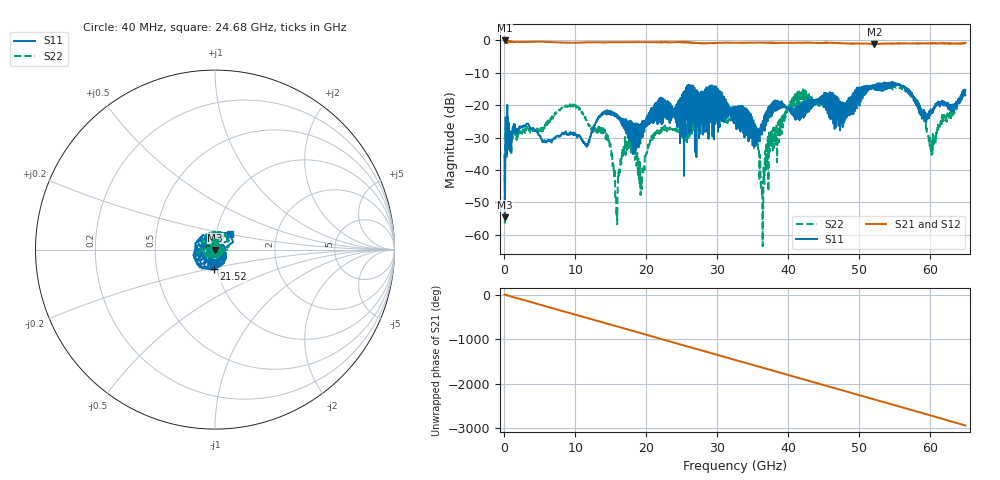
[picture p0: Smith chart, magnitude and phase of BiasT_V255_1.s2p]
! Created Tue Jul 15 19:49:57 2008
# hz S ma R 50
! 2 Port Network Data from blockName block
! freq  magS11  angS11  magS21  angS21  magS12  angS12  magS22  angS22
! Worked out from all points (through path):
!   1601 points, 40 MHz to 65 GHz, reference 50 ohm
!   highest |S21| = -0.03 dB at 80.6 MHz (marker M1); lowest = -1.1 dB at 52.17 GHz (marker M2)
!   group delay of S21, straight-line fit = 125 ps
!   lowest |S11| = -54.7 dB at 80.6 MHz (marker M3), VSWR 1.00, Z = 50.1 - j0.149 ohm
!   |S11| at or under -10 dB: start of sweep to end of sweep
!   |S22| runs from -63.5 to -13.2 dB; largest |S21 - S12| = 0.05
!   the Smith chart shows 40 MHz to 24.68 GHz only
!   S11 on the Smith chart (normalised r, x): 40 MHz: 1.00, +0.03; 21.52 GHz: 0.96, -0.21; 24.68 GHz: 1.16, +0.21
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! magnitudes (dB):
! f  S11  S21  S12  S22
! 40 MHz  -35.6  -0.1  -0.1  -35.2
! 80.6 MHz  -54.7  0.0  0.0  -56.9
! 3.085 GHz  -26.0  -0.5  -0.5  -27.5
! 10.88 GHz  -30.3  -0.7  -0.7  -21.8
! 14.45 GHz  -22.2  -0.6  -0.6  -30.7
! 15.75 GHz  -23.6  -0.6  -0.6  -48.2
! 17.09 GHz  -25.5  -0.6  -0.5  -35.4
! 19.32 GHz  -30.2  -0.5  -0.5  -42.5
! 21.52 GHz  -19.2  -0.6  -0.5  -28.0
! 21.72 GHz  -19.0  -0.6  -0.5  -27.7
! 24.68 GHz  -18.3  -0.6  -0.5  -27.9
! 32.52 GHz  -25.5  -0.7  -0.8  -22.8
! 35.2 GHz  -33.2  -0.7  -0.7  -27.8
! 36.38 GHz  -27.0  -0.7  -0.7  -46.5
! 37.64 GHz  -21.4  -0.8  -0.7  -32.6
! 40.23 GHz  -21.3  -0.8  -0.7  -21.3
! 43.36 GHz  -20.4  -0.7  -0.7  -17.6
! 52.17 GHz  -13.9  -1.1  -1.2  -14.2
! 54.2 GHz  -13.6  -1.0  -1.0  -14.1
! 58.02 GHz  -18.1  -1.0  -1.0  -19.4
! 60.29 GHz  -21.5  -1.0  -0.9  -31.0
! 65 GHz  -17.0  -0.8  -1.2  -14.9
